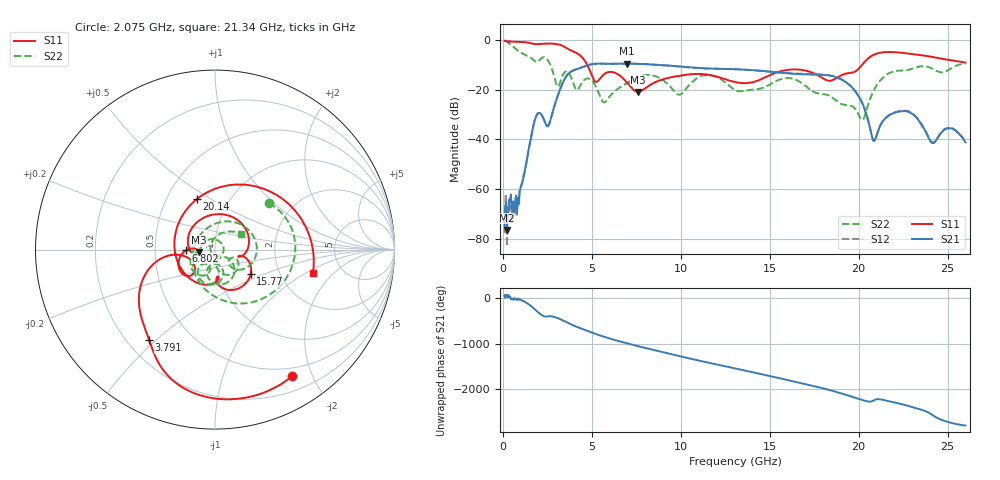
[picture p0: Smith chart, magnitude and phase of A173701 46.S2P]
!  2-Port S-parameters saved by WinCal
! VAR MeasName=S-Parameters (CALIBRATED_DATA) read from VNA (N5245A)
! VAR MeasDate=2017-6-7 10:31:28
! VAR NAME=A173701 46
! VAR FILENAME=A173701 46.S2P
! VAR DATE=2017-6-7 10:31:28
! VAR PHYS_PORTS=1,2
# Hz S DB R 50
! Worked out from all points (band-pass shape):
!   801 points, 100 MHz to 26 GHz, reference 50 ohm
!   highest |S21| = -9.52 dB at 6.996 GHz (marker M1); lowest = -76.4 dB at 229.5 MHz (marker M2)
!   |S21| within 3 dB of the highest: 3.896 GHz to 14.7 GHz (10.81 GHz wide, 116 % of centre)
!   lowest |S11| = -20.9 dB at 7.611 GHz (marker M3), VSWR 1.20, Z = 41.8 - j1.31 ohm
!   |S11| at or under -10 dB: 4.74 GHz to 20.2 GHz (15.46 GHz wide, 124 % of centre)
!   |S22| runs from -32.2 to -0.2 dB; largest |S21 - S12| = 0.0048
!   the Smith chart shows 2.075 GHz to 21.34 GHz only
!   S11 on the Smith chart (normalised r, x): 2.075 GHz: 0.38, -1.72; 3.791 GHz: 0.29, -0.47; 6.802 GHz: 0.72, -0.01; 15.77 GHz: 1.42, -0.42; 20.14 GHz: 0.70, +0.43; 21.34 GHz: 3.07, -1.16
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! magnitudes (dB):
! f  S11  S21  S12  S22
! 100 MHz  -0.3  -74.5  -77.6  -0.2
! 229.5 MHz  -0.6  -76.4  -82.9  -0.7
! 779.9 MHz  -0.7  -69.7  -70.2  -3.9
! 2.075 GHz  -1.6  -29.5  -29.5  -8.0
! 2.561 GHz  -1.5  -34.4  -34.4  -8.5
! 3.079 GHz  -1.8  -22.6  -22.5  -18.8
! 3.791 GHz  -4.1  -13.0  -12.9  -14.3
! 4.438 GHz  -6.9  -11.0  -11.0  -17.4
! 5.701 GHz  -13.7  -9.6  -9.6  -25.1
! 6.802 GHz  -15.8  -9.5  -9.5  -18.1
! 6.996 GHz  -17.3  -9.5  -9.5  -17.2
! 7.611 GHz  -20.9  -9.6  -9.6  -14.9
! 8.744 GHz  -16.5  -10.0  -10.1  -15.1
! 9.877 GHz  -14.5  -10.6  -10.7  -22.0
! 13.05 GHz  -16.9  -11.8  -11.8  -20.2
! 15.77 GHz  -12.3  -13.3  -13.2  -15.5
! 17.39 GHz  -13.1  -14.0  -13.8  -20.5
! 20.14 GHz  -10.5  -24.4  -24.6  -31.9
! 20.82 GHz  -6.1  -40.4  -40.3  -20.8
! 21.34 GHz  -5.0  -32.9  -32.8  -15.4
! 21.69 GHz  -4.9  -30.4  -30.3  -13.5
! 26 GHz  -9.1  -41.2  -41.0  -9.5
